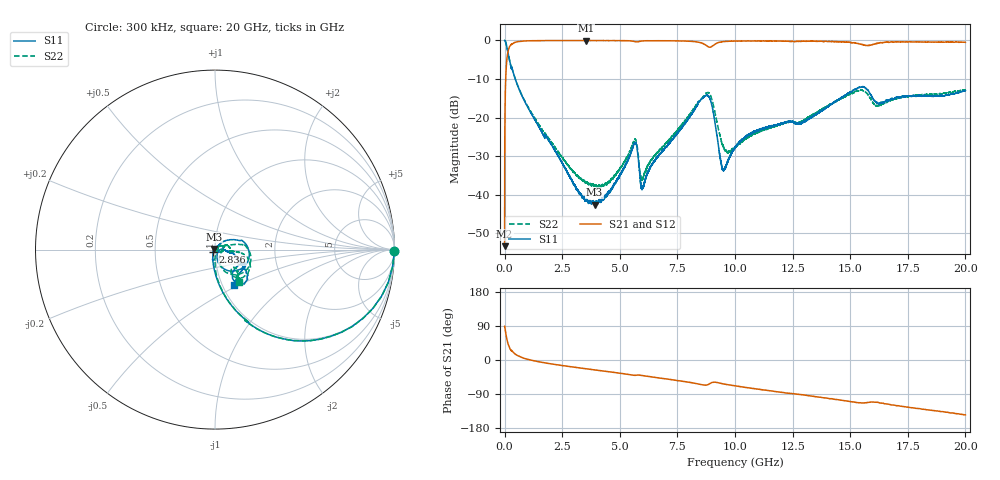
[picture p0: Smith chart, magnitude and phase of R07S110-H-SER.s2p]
!{R07S110}
!Johanson Technology Inc.
!www.johansontechnology.com
!Test Board Conditions:
!Substrate Type  RO4350B
!Substrate Thickness  10 mil
!Substrate Dk  3.66
!TL Type: GCPW
!TL Trace Width  21 mil
!TL Gap  20 mil
!Electrode orientation  Horizontal
!DUT TOPOLOGY	SERIES
!Mounting Pad LxW  16x21 mil
! Created Sat Feb  6 11:44:00 2021
# hz S ma R 50
! 2 Port Network Data from SP1.SP block
! freq  magS11  angS11  magS21  angS21  magS12  angS12  magS22  angS22
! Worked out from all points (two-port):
!   20001 points, 300 kHz to 20 GHz, reference 50 ohm
!   highest |S21| = -0.02 dB at 3.527 GHz (marker M1); lowest = -53.4 dB at 300 kHz (marker M2)
!   |S21| within 3 dB of the highest: 143.4 MHz to end of sweep
!   lowest |S11| = -42.6 dB at 3.906 GHz (marker M3), VSWR 1.01, Z = 49.4 + j0.4 ohm
!   |S11| at or under -10 dB: 461.9 MHz to end of sweep
!   |S22| runs from -38.2 to 0.0 dB; largest |S21 - S12| = 0.013
!   S11 on the Smith chart (normalised r, x): 300 kHz: open; 2.836 GHz: 0.98, -0.03; 20 GHz: 1.14, -0.47
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300000  1 -0.4  0.002138 89.2  0.002113 88.7  0.9987 -0.4
1.063e8  0.7997 -37.5  0.5956 52.9  0.5966 52.8  0.8008 -37.4
2.373e8  0.5129 -61.0  0.8545 29.4  0.8529 29.4  0.5133 -61.1
7.793e8  0.1846 -84.3  0.9814 5.9  0.9807 5.9  0.187 -83.4
2.8363e9  0.01668 -130.0  0.9968 -17.4  0.9965 -17.4  0.02223 -75.5
3.3343e9  0.009634 -162.7  0.9968 -21.5  0.9969 -21.5  0.01567 -53.9
3.5273e9  0.008369 -179.6  0.9976 -23.1  0.9961 -23.0  0.01439 -46.7
3.9063e9  0.007414 146.9  0.9956 -26.1  0.9964 -26.1  0.01285 -24.9
4.6353e9  0.01183 86.7  0.9948 -31.9  0.9958 -31.9  0.0159 19.8
5.6343e9  0.04592 18.1  0.9679 -40.5  0.9684 -40.4  0.05091 16.5
5.9853e9  0.01211 11.6  0.9863 -41.1  0.9872 -41.1  0.01595 15.4
6.6673e9  0.03154 47.5  0.9921 -47.1  0.9922 -47.1  0.03547 34.6
8.8053e9  0.1946 -19.0  0.8406 -65.5  0.8396 -65.6  0.2106 -22.7
9.0193e9  0.1338 -59.5  0.8464 -59.0  0.8461 -59.0  0.1623 -57.8
9.4723e9  0.0214 -40.6  0.9622 -62.8  0.9631 -62.8  0.04383 -53.4
1.00003e10  0.04057 3.2  0.9826 -68.4  0.9816 -68.4  0.0415 1.8
1.08903e10  0.0658 -8.0  0.986 -76.1  0.9836 -76.0  0.06279 21.4
1.33343e10  0.1012 -11.2  0.9762 -95.2  0.9773 -95.3  0.1056 -5.2
1.54553e10  0.2457 -44.7  0.8952 -113.0  0.8934 -113.1  0.2262 -35.4
1.61313e10  0.1573 -48.8  0.9115 -111.6  0.9102 -111.5  0.1427 -49.8
1.66673e10  0.1656 -27.7  0.9449 -116.7  0.9496 -117.0  0.1642 -42.2
2e10  0.224 -61.4  0.9491 -144.9  0.9479 -144.7  0.2275 -53.1
